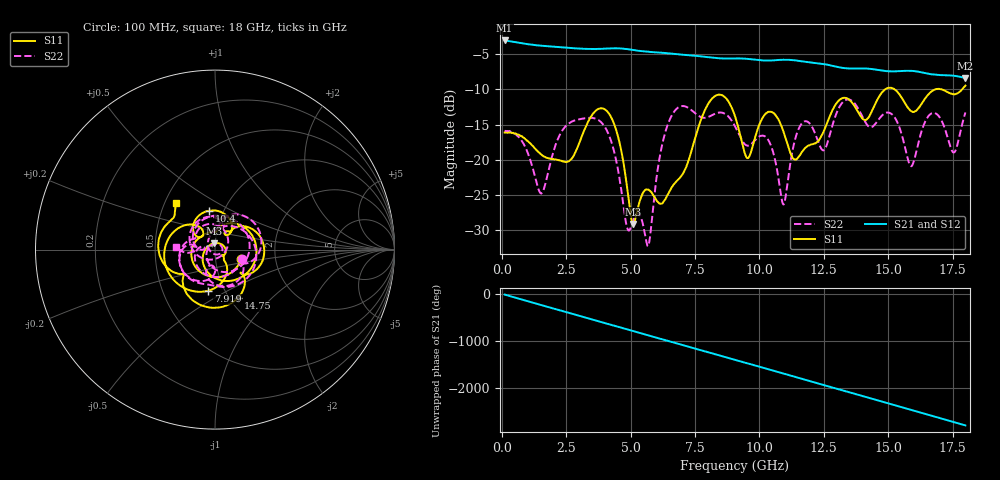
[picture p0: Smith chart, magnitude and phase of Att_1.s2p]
#  HZ  S  DB  R  50.00
! Rohde & Schwarz Vector Network Analyzer
! Rohde-Schwarz,ZNB40-4Port,1311601084101679,3.45
! Created: UTC 4/25/2025, 8:42:17 AM
! freq[Hz]  db:S11  ang:S11  db:S21  ang:S21  db:S12  ang:S12  db:S22  ang:S22
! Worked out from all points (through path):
!   1750 points, 100 MHz to 18 GHz, reference 50 ohm
!   highest |S21| = -3.09 dB at 100 MHz (marker M1); lowest = -8.4 dB at 18 GHz (marker M2)
!   group delay of S21, straight-line fit = 428 ps
!   lowest |S11| = -29.1 dB at 5.105 GHz (marker M3), VSWR 1.07, Z = 49.2 + j3.39 ohm
!   |S11| at or under -10 dB: start of sweep to 14.89 GHz; 15.24 GHz to 16.85 GHz (1.61 GHz wide, 10 % of centre); 17.03 GHz to 17.88 GHz (844.1 MHz wide, 4.84 % of centre)
!   |S22| runs from -32.2 to -11.4 dB; largest |S21 - S12| = 0.00098
!   S11 on the Smith chart (normalised r, x): 100 MHz: 1.34, -0.14; 7.919 GHz: 0.84, -0.41; 10.4 GHz: 0.86, +0.39; 14.75 GHz: 1.09, -0.65; 18 GHz: 0.58, +0.33
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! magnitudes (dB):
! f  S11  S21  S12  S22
! 100 MHz  -16.1  -3.1  -3.1  -15.9
! 1.523 GHz  -19.3  -3.8  -3.8  -24.8
! 3.088 GHz  -16.8  -4.3  -4.3  -14.2
! 4.194 GHz  -13.7  -4.2  -4.2  -16.9
! 4.849 GHz  -23.6  -4.3  -4.3  -29.5
! 5.105 GHz  -29.1  -4.5  -4.5  -28.5
! 5.688 GHz  -24.2  -4.7  -4.7  -32.2
! 6.067 GHz  -26.0  -4.8  -4.8  -20.9
! 6.763 GHz  -23.1  -5.0  -5.0  -12.8
! 7.919 GHz  -12.7  -5.4  -5.4  -14.0
! 9.055 GHz  -13.9  -5.6  -5.6  -15.3
! 9.546 GHz  -19.8  -5.7  -5.7  -18.0
! 10.4 GHz  -13.2  -5.9  -5.9  -17.6
! 10.94 GHz  -16.1  -5.8  -5.8  -26.3
! 11.48 GHz  -19.8  -6.0  -6.0  -16.0
! 12.04 GHz  -17.8  -6.2  -6.2  -15.4
! 14.75 GHz  -10.5  -7.4  -7.4  -13.8
! 15.02 GHz  -9.8  -7.5  -7.5  -13.3
! 15.89 GHz  -13.1  -7.4  -7.4  -20.9
! 16.62 GHz  -10.5  -7.9  -7.8  -13.6
! 17.55 GHz  -10.7  -8.1  -8.1  -19.0
! 18 GHz  -9.5  -8.4  -8.4  -13.3
